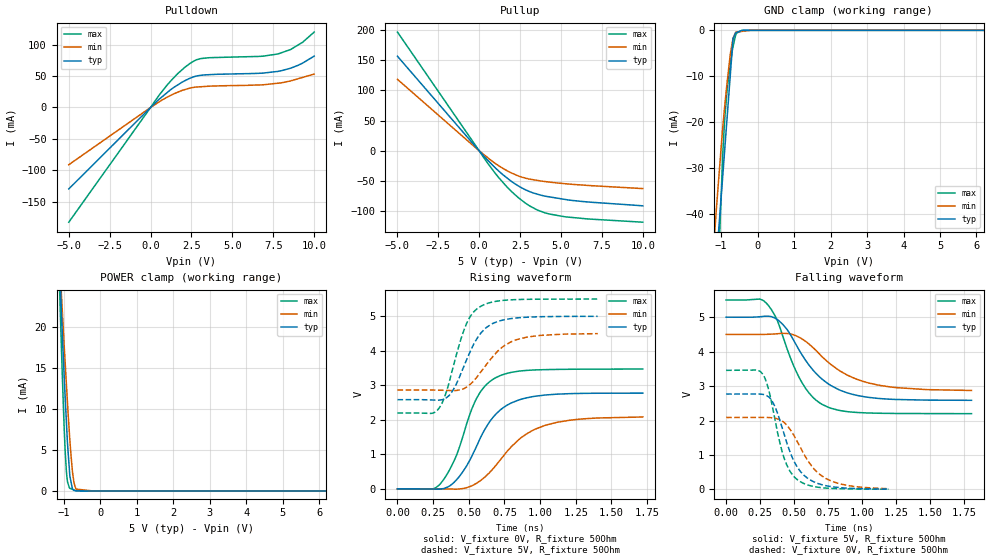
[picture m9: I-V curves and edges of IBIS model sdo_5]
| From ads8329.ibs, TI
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|   sdo_5 Model
[Model]   sdo_5
Model_type   3-state
Polarity   Non-Inverting
Vmeas = 2.5
Vref = 2.5
Cref = 30pF
Rref = 50
|   typ   min   max
|   (nom PVT)   (Fast PVT)   (slow PVT)
|C_comp from frequency sweep method(F=0.05MHz)
|C_comp   4.863e-11   1.707e-11   1.282e-10
|ON state : BUFFER OUTPUT TURNED HIGH
|C_comp   4.863e-11   1.707e-11   1.282e-10
|OFF state: BUFFER IN HIGH IMPEDANCE
|C_comp   3.729e-12   3.906e-12   3.570e-12
|C_comp from LC tank measurement(L=1nH)
C_comp   2.9805e-12  2.730e-12   3.131e-12
|OFF state: BUFFER IN HIGH IMPEDANCE
|Resonant Frequency(Hz)   3.000e+09   3.120e+09   2.940e+09
|C_comp   2.817e-12   2.605e-12   2.933e-12
|ON state : BUFFER OUTPUT TURNED HIGH
|Resonant Frequency(Hz)   2.840e+09   2.980e+09   2.760e+09
|C_comp   3.144e-12   2.855e-12   3.329e-12
| Where nom  PVT is Nominal Process,  5V,  28C
|   Fast PVT is Strong Process,   5.5V,  -40C
|   Slow PVT is Weak Process,   4.5V,  88C
[Voltage Range]   5   4.5   5.5
|Ambient Temperature   25   85   -40
|Junction Temperature
[Temperature Range]   28   88   -40
[Pullup Reference]   5   4.5   5.5
[Pulldown Reference]   0   0   0
[Power Clamp Reference]   5   4.5   5.5
[GND Clamp Reference]   0   0   0
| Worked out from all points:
|   slope of the pulldown table from 0 to 0.75 V, typ, clamps not added: 41.6 ohm
|   slope of the pullup table from 0 to 0.75 V, typ, clamps not added: 34.4 ohm
|   GND clamp passes 1 mA (typ) near -0.63 V on its own axis
|   POWER clamp passes 1 mA (typ) near -0.80 V on its own axis
|   falling waveform, V_fixture 5V, R_fixture 50Ohm: 20-80 % time 280ps typ, 338ps min, 215ps max; typ from 5 V to 2.59 V
|   rising waveform, V_fixture 0V, R_fixture 50Ohm: 20-80 % time 236ps typ, 304ps min, 193ps max; typ from 0 V to 2.77 V
|   rising waveform, V_fixture 5V, R_fixture 50Ohm: 20-80 % time 169ps typ, 211ps min, 144ps max; typ from 2.58 V to 5 V
|   falling waveform, V_fixture 0V, R_fixture 50Ohm: 20-80 % time 161ps typ, 208ps min, 127ps max; typ from 2.77 V to 0.009 V
[Pulldown]
|   Voltage   I(typ)   I(min)   I(max)
-5V       -129.7mA   -91.16mA   -182.7mA
544.5mV   13.56mA    9.392mA    20.29mA
1.27V     29.15mA    19.86mA    43.43mA
2.084V    42.51mA    28.38mA    63.78mA
2.574V    48.25mA    31.78mA    72.91mA
3.08V     51.29mA    33.04mA    77.94mA
6.6V      54.42mA    35.87mA    81.3mA
7.788V    57.5mA     38.68mA    85.29mA
8.563V    62.61mA    42.36mA    92.36mA
9.28V     70.47mA    47.78mA    103.6mA
10V       81.79mA    53.22mA    120.1mA
[GND Clamp]
|   Voltage   I(typ)   I(min)   I(max)
-5V       -897.3mA   -658.7mA   -1.295A
-1.238V   -68.2mA    -51.34mA   -96.17mA
-1.143V   -51.64mA   -40.1mA    -70.51mA
-1.028V   -39.31mA   -28.37mA   -41.82mA
-957mV    -31.74mA   -21.13mA   -27.29mA
-891mV    -24.74mA   -15.56mA   -18.12mA
-814mV    -16.59mA   -9.738mA   -11.5mA
-742.5mV  -9.016mA   -4.846mA   -6.946mA
-675mV    -1.867mA   -1.787mA   -3.58mA
-598.5mV  -555.5uA   -394.5uA   -973.7uA
-407mV    -7.391uA   -203.8uA   -2.213uA
10V       0A         0A         0A
[Pullup]
|   Voltage   I(typ)   I(min)   I(max)
-5V       156.7mA    118.4mA    196.7mA
456.5mV   -13.76mA   -9.979mA   -18.22mA
1.166V    -32.83mA   -24.21mA   -43.49mA
1.672V    -44.32mA   -32.44mA   -59.07mA
2.376V    -57.83mA   -41.4mA    -77.2mA
3.08V     -67.48mA   -46.84mA   -91.12mA
3.526V    -71.47mA   -48.82mA   -97.64mA
4.268V    -76.1mA    -51.66mA   -104.5mA
5.192V    -80.22mA   -54.24mA   -109mA
6.6V      -84.52mA   -57.17mA   -112.6mA
10V       -91.03mA   -62.47mA   -118.1mA
[POWER Clamp]
|   Voltage   I(typ)   I(min)   I(max)
-5V       207.8mA    188.7mA    235.2mA
-1.14V    29.99mA    30.26mA    28.19mA
-1.105V   26.12mA    27.21mA    23.03mA
-1.098V   25.28mA    26.55mA    21.95mA
-1.045V   19.51mA    22.19mA    14.5mA
-990mV    13.86mA    17.67mA    7.634mA
-929.5mV  8.415mA    12.99mA    2.38mA
-835mV    1.831mA    6.223mA    318.2uA
-720mV    60.44uA    951.4uA    122.3uA
-666mV    12.23uA    221.7uA    30.32uA
-202.5mV  0A         0A         427.1nA
10V       0A         0A         0A
[Ramp]
R_load = 50
|   typ   min   max
dV/dt_r   1.6665/2.35957e-10   1.25437/3.06262e-10   2.08344/1.93637e-10
dV/dt_f   1.45014/2.8107e-10   0.982492/3.42727e-10   1.98164/2.15429e-10
[Falling Waveform]
V_fixture = 5V
V_fixture_min = 4.5V
V_fixture_max = 5.5V
R_fixture = 50Ohm
|   Time   V(typ)   V(min)   V(max)
0s        5V         4.5V       5.5V
296ps     5.029V     4.502V     5.407V
366ps     4.957V     4.516V     4.988V
420ps     4.775V     4.532V     4.411V
558ps     3.907V     4.37V      3.099V
646ps     3.433V     4.091V     2.644V
750ps     3.067V     3.694V     2.386V
924ps     2.765V     3.258V     2.245V
1.112ns   2.644V     3.034V     2.212V
1.804ns   2.587V     2.872V     2.2V
[Rising Waveform]
V_fixture = 0V
V_fixture_min = 0V
V_fixture_max = 0V
R_fixture = 50Ohm
|   Time   V(typ)   V(min)   V(max)
0s        1.719nV    1.915nV    1.479nV
242ps     -3.637mV   628.1uV    -5.3mV
302ps     -5.598mV   -960.1uV   152.7mV
424ps     307.5mV    -7.257mV   1.082V
554ps     1.226V     160.5mV    2.615V
618ps     1.759V     361mV      2.995V
696ps     2.189V     711.1mV    3.234V
864ps     2.591V     1.47V      3.415V
1.038ns   2.718V     1.842V     3.453V
1.72ns    2.772V     2.081V     3.469V
[Rising Waveform]
V_fixture = 5V
V_fixture_min = 4.5V
V_fixture_max = 5.5V
R_fixture = 50Ohm
|   Time   V(typ)   V(min)   V(max)
0s        2.582V     2.861V     2.196V
236ps     2.575V     2.861V     2.185V
288ps     2.567V     2.858V     2.318V
328ps     2.601V     2.853V     2.634V
378ps     2.784V     2.847V     3.338V
484ps     3.731V     2.946V     4.782V
584ps     4.509V     3.384V     5.288V
704ps     4.849V     3.994V     5.44V
832ps     4.949V     4.316V     5.482V
1.404ns   4.997V     4.495V     5.497V
[Falling Waveform]
V_fixture = 0V
V_fixture_min = 0V
V_fixture_max = 0V
R_fixture = 50Ohm
|   Time   V(typ)   V(min)   V(max)
0s        2.769V     2.088V     3.457V
274ps     2.757V     2.09V      3.32V
308ps     2.698V     2.088V     2.964V
350ps     2.478V     2.073V     2.213V
424ps     1.64V      1.951V     938.9mV
470ps     1.088V     1.744V     525.7mV
530ps     609.7mV    1.337V     263.9mV
640ps     230.1mV    622.7mV    88.08mV
754ps     92.88mV    276.6mV    33.52mV
1.194ns   9.497mV    20.59mV    7.135mV
